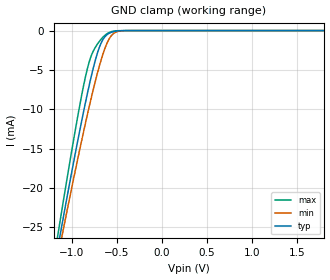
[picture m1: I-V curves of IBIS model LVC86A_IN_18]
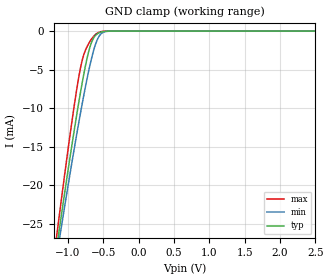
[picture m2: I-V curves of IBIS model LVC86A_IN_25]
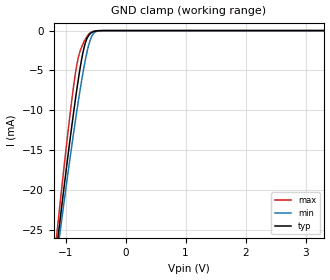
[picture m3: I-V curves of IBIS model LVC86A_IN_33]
| Texas Instruments Incorporated
| QUADRUPLE 2-INPUT EXCLUSIVE-OR GATES
| Marketing part#   Voltage Range   Package-type   #pins/pkg drawing
| SN74LVC86AD   1.65V - 3.6V   SOIC   14-pin D
| SN74LVC86ADB   1.65V - 3.6V   SSOP   14-pin DB
| SN74LVC86ANS   1.65V - 3.6V   SO   14-pin NS
| SN74LVC86APW   1.65V - 3.6V   TSSOP   14-pin PW
| SN74LVC86ARGY   1.65V - 3.6V   VQFN   14-pin RGY
[IBIS Ver]   3.2
[Comment char]  |_char
[File Name]   sn74lvc86a.ibs
[File Rev]   1.2 | k_die
[Date]   January 3, 2012
[Source]   Model built from TISPICE simulations at:
   Texas Instruments Incorporated, SLL
   Continuing support by
   Webench Design Center
   12500 TI Blvd
   Dallas, TX -75243
   For Support e-mail: elab_ibis@list.ti.com
[Notes]   Revision History
   Rev 1.1: 06/27/2002
   Rev 1.2: 01/03/2012  Added QFN package component
[Disclaimer] This product is designed as an aid for customers of Texas
   Instruments.
   No warranties, either expressed or implied, with respect
   to this third party software (if any) or with respect to
   its fitness for any particular purpose is claimed by Texas
   Instruments or the author. The software (if any) is provided
   solely on an "as is" basis. The entire risk as to its quality
   and performance is with the customer
[Copyright]   (C)Copyright 2011 Texas Instruments Incorporated.
   All rights reserved.
| Component LVC86A_D 14-pin SOIC
[Component]   LVC86A_D
[Manufacturer]  Texas Instruments, Inc.
[Package]
|   typ   min   max
R_pkg   3.100e-02   2.800e-02   3.400e-02
L_pkg   3.109e-09   2.462e-09   3.889e-09
C_pkg   4.730e-13   3.630e-13   6.280e-13
[Pin]   signal_name   model_name   R_pin   L_pin   C_pin
1   1A   LVC86A_IN   3.300e-02   3.854e-09   6.220e-13
2   1B   LVC86A_IN   3.200e-02   3.188e-09   4.730e-13
3   1Y   LVC86A_OUT   2.800e-02   2.462e-09   3.770e-13
4   2A   LVC86A_IN   3.100e-02   2.596e-09   3.630e-13
5   2B   LVC86A_IN   2.800e-02   2.521e-09   3.720e-13
6   2Y   LVC86A_OUT   3.400e-02   3.250e-09   4.760e-13
7   GND   GND   3.400e-02   3.889e-09   6.280e-13
8   3Y   LVC86A_OUT   3.400e-02   3.889e-09   6.280e-13
9   3A   LVC86A_IN   3.400e-02   3.250e-09   4.760e-13
10   3B   LVC86A_IN   2.800e-02   2.521e-09   3.720e-13
11   4Y   LVC86A_OUT   3.100e-02   2.596e-09   3.640e-13
12   4A   LVC86A_IN   2.800e-02   2.462e-09   3.770e-13
13   4B   LVC86A_IN   3.200e-02   3.188e-09   4.730e-13
14   VCC   POWER   3.300e-02   3.854e-09   6.220e-13
| Component LVC86A_DB 14-pin SSOP
[Component]   LVC86A_DB
[Manufacturer]  Texas Instruments, Inc.
[Package]
|   typ   min   max
R_pkg   4.400e-02   4.100e-02   4.600e-02
L_pkg   3.551e-09   3.258e-09   3.927e-09
C_pkg   4.020e-13   3.600e-13   4.210e-13
[Pin]   signal_name   model_name   R_pin   L_pin   C_pin
1   1A   LVC86A_IN   4.600e-02   3.927e-09   4.080e-13
2   1B   LVC86A_IN   4.400e-02   3.587e-09   4.210e-13
3   1Y   LVC86A_OUT   4.100e-02   3.289e-09   3.980e-13
4   2A   LVC86A_IN   4.200e-02   3.258e-09   3.600e-13
5   2B   LVC86A_IN   4.100e-02   3.286e-09   4.030e-13
6   2Y   LVC86A_OUT   4.400e-02   3.586e-09   4.210e-13
7   GND   GND   4.600e-02   3.927e-09   4.080e-13
8   3Y   LVC86A_OUT   4.600e-02   3.927e-09   4.080e-13
9   3A   LVC86A_IN   4.400e-02   3.586e-09   4.210e-13
10   3B   LVC86A_IN   4.100e-02   3.286e-09   4.030e-13
11   4Y   LVC86A_OUT   4.300e-02   3.258e-09   3.600e-13
12   4A   LVC86A_IN   4.100e-02   3.289e-09   3.980e-13
13   4B   LVC86A_IN   4.400e-02   3.587e-09   4.210e-13
14   VCC   POWER   4.600e-02   3.927e-09   4.080e-13
| Component LVC86A_NS 14-pin SOP
[Component]   LVC86A_NS
[Manufacturer]  Texas Instruments, Inc.
[Package]
|   typ   min   max
R_pkg   4.500e-02   3.900e-02   5.400e-02
L_pkg   3.796e-09   2.561e-09   4.952e-09
C_pkg   5.280e-13   2.880e-13   7.100e-13
[Pin]   signal_name   model_name   R_pin   L_pin   C_pin
1   1A   LVC86A_IN   4.700e-02   4.867e-09   7.060e-13
2   1B   LVC86A_IN   5.100e-02   4.083e-09   5.920e-13
3   1Y   LVC86A_OUT   4.100e-02   2.915e-09   3.760e-13
4   2A   LVC86A_IN   3.900e-02   2.561e-09   2.880e-13
5   2B   LVC86A_IN   4.100e-02   3.101e-09   4.300e-13
6   2Y   LVC86A_OUT   4.700e-02   4.047e-09   5.890e-13
7   GND   GND   5.100e-02   4.909e-09   7.000e-13
8   3Y   LVC86A_OUT   4.500e-02   4.784e-09   6.940e-13
9   3A   LVC86A_IN   5.400e-02   4.176e-09   5.970e-13
10   3B   LVC86A_IN   3.900e-02   3.287e-09   4.490e-13
11   4Y   LVC86A_OUT   3.900e-02   2.586e-09   2.940e-13
12   4A   LVC86A_IN   4.000e-02   2.802e-09   3.710e-13
13   4B   LVC86A_IN   4.900e-02   4.080e-09   5.930e-13
14   VCC   POWER   5.200e-02   4.952e-09   7.100e-13
| Component LVC86A_PW 14-pin TSSOP
[Component]   LVC86A_PW
[Manufacturer]  Texas Instruments, Inc.
[Package]
|   typ   min   max
R_pkg   3.200e-02   2.900e-02   3.500e-02
L_pkg   2.378e-09   2.170e-09   2.680e-09
C_pkg   3.140e-13   2.700e-13   3.350e-13
[Pin]   signal_name   model_name   R_pin   L_pin   C_pin
1   1A   LVC86A_IN   3.300e-02   2.618e-09   3.300e-13
2   1B   LVC86A_IN   3.100e-02   2.313e-09   3.170e-13
3   1Y   LVC86A_OUT   3.000e-02   2.310e-09   3.140e-13
4   2A   LVC86A_IN   3.100e-02   2.173e-09   2.720e-13
5   2B   LVC86A_IN   3.000e-02   2.204e-09   3.090e-13
6   2Y   LVC86A_OUT   3.200e-02   2.315e-09   3.170e-13
7   GND   GND   3.500e-02   2.680e-09   3.350e-13
8   3Y   LVC86A_OUT   3.300e-02   2.640e-09   3.330e-13
9   3A   LVC86A_IN   3.400e-02   2.347e-09   3.190e-13
10   3B   LVC86A_IN   2.900e-02   2.277e-09   3.130e-13
11   4Y   LVC86A_OUT   3.100e-02   2.170e-09   2.700e-13
12   4A   LVC86A_IN   3.100e-02   2.244e-09   3.110e-13
13   4B   LVC86A_IN   3.300e-02   2.343e-09   3.210e-13
14   VCC   POWER   3.500e-02   2.657e-09   3.320e-13
| Component LVC86A_RGY 14-pin QFN
[Component]   LVC86A_RGY
[Manufacturer]  Texas Instruments, Inc.
[Package]
|   typ   min   max
R_pkg   0.07867   0.07388   0.08515
L_pkg   1.5346n   1.43869n   1.67414n
C_pkg   0.14715p   0.11801p   0.16038p
[Pin]   signal_name   model_name   R_pin   L_pin   C_pin
1   1A   LVC86A_IN   0.07388   1.43869n   0.12600p
2   1B   LVC86A_IN   0.08264   1.62504n   0.15219p
3   1Y   LVC86A_OUT   0.07686   1.49770n   0.15790p
4   2A   LVC86A_IN   0.07508   1.45913n   0.15548p
5   2B   LVC86A_IN   0.07847   1.53230n   0.16038p
6   2Y   LVC86A_OUT   0.08492   1.67414n   0.15346p
7   GND   GND   0.07730   1.51242n   0.12786p
8   3Y   LVC86A_OUT   0.07653   1.49122n   0.12936p
9   3A   LVC86A_IN   0.08515   1.67034n   0.15559p
10   3B   LVC86A_IN   0.07816   1.51600n   0.15984p
11   4Y   LVC86A_OUT   0.07551   1.45843n   0.15613p
12   4A   LVC86A_IN   0.07676   1.48590n   0.15722p
13   4B   LVC86A_IN   0.08290   1.62154n   0.15063p
14   VCC   POWER   0.07724   1.50154n   0.11801p
| Model LVC86A_IN
[Model Selector]   LVC86A_IN
LVC86A_IN_18   1.8 volt Vcc
LVC86A_IN_25   2.5 volt Vcc
LVC86A_IN_33   3.3 volt Vcc
| Model LVC86A_OUT
[Model Selector]   LVC86A_OUT
LVC86A_OUT_18   1.8 volt Vcc
LVC86A_OUT_25   2.5 volt Vcc
LVC86A_OUT_33   3.3 volt Vcc
| Models and submodels in the file (6): LVC86A_IN_18 (Input), LVC86A_IN_25 (Input), LVC86A_IN_33 (Input), LVC86A_OUT_18 (Output), LVC86A_OUT_25 (Output), LVC86A_OUT_33 (Output)
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[Model]   LVC86A_IN_18
Model_type  Input
Vinl=0.5775
Vinh=1.2675
| variable   typ   min   max
C_comp   2.65pF   2.20pF   3.15pF
[Temperature Range]   40   100   -40
| Ambient temperature   25   85   -40
[Voltage range]   1.8   1.65   1.95
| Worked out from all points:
|   GND clamp passes 1 mA (typ) near -0.64 V on its own axis
[GND Clamp]
| LVC86A_IN_18
|   Voltage   I(typ)   I(min)   I(max)
-5.5V     -338.9mA   -314.3mA   -369mA
-1.16V    -28.09mA   -29.24mA   -26.56mA
-1.12V    -25.56mA   -26.92mA   -23.71mA
-1.085V   -23.36mA   -24.91mA   -21.25mA
-925mV    -13.65mA   -15.98mA   -10.52mA
-820mV    -7.797mA   -10.48mA   -4.654mA
-770mV    -5.293mA   -8.026mA   -2.891mA
-695mV    -2.253mA   -4.666mA   -1.432mA
-600mV    -473.7uA   -1.449mA   -358.4uA
-535mV    -136.2uA   -379.8uA   -78.5uA
-445mV    -16.2uA    -36.49uA   -4.833uA
1.8V      41.95pA    147.4pA    23.47pA
[Model]   LVC86A_IN_25
Model_type  Input
Vinl=0.7
Vinh=1.7
| variable   typ   min   max
C_comp   2.57pF   2.04pF   3.21pF
[Temperature Range]   40   100   -40
| Ambient temperature   25   85   -40
[Voltage range]   2.5   2.3   2.7
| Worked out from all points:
|   GND clamp passes 1 mA (typ) near -0.64 V on its own axis
[GND Clamp]
| LVC86A_IN_25
|   Voltage   I(typ)   I(min)   I(max)
-5.5V     -338.9mA   -314.3mA   -369mA
-1.17V    -28.73mA   -29.82mA   -27.27mA
-1.13V    -26.19mA   -27.5mA    -24.42mA
-1.095V   -23.98mA   -25.48mA   -21.95mA
-925mV    -13.65mA   -15.98mA   -10.52mA
-825mV    -8.06mA    -10.74mA   -4.88mA
-775mV    -5.531mA   -8.266mA   -3.027mA
-700mV    -2.416mA   -4.874mA   -1.51mA
-590mV    -396.4uA   -1.217mA   -293.2uA
-515mV    -88.16uA   -231.8uA   -44.89uA
-395mV    -4.232uA   -9.445uA   -775nA
2.5V      57.25pA    176.8pA    32.61pA
[Model]   LVC86A_IN_33
Model_type  Input
Vinl=0.8
Vinh=2.0
| variable   typ   min   max
C_comp   2.50pF   1.92pF   3.13pF
[Temperature Range]   40   100   -40
| Ambient temperature   25   85   -40
[Voltage range]   3.3   3   3.6
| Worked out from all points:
|   GND clamp passes 1 mA (typ) near -0.64 V on its own axis
[GND Clamp]
| LVC86A_IN_33
|   Voltage   I(typ)   I(min)   I(max)
-5.5V     -338.9mA   -314.3mA   -369mA
-1.14V    -26.82mA   -28.07mA   -25.13mA
-1.105V   -24.61mA   -26.05mA   -22.65mA
-1.075V   -22.73mA   -24.34mA   -20.55mA
-915mV    -13.07mA   -15.45mA   -9.893mA
-860mV    -9.954mA   -12.53mA   -6.658mA
-805mV    -7.019mA   -9.733mA   -4.027mA
-730mV    -3.528mA   -6.174mA   -2.02mA
-665mV    -1.428mA   -3.486mA   -1.009mA
-585mV    -362.1uA   -1.111mA   -263.9uA
-510mV    -78.77uA   -204.1uA   -38.82uA
3.3V      76.2pA     212.8pA    43.07pA
